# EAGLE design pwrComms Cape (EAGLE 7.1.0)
CNAME: Bristol Community College; CREVISION: v1r0; DESIGNER: J. Brian
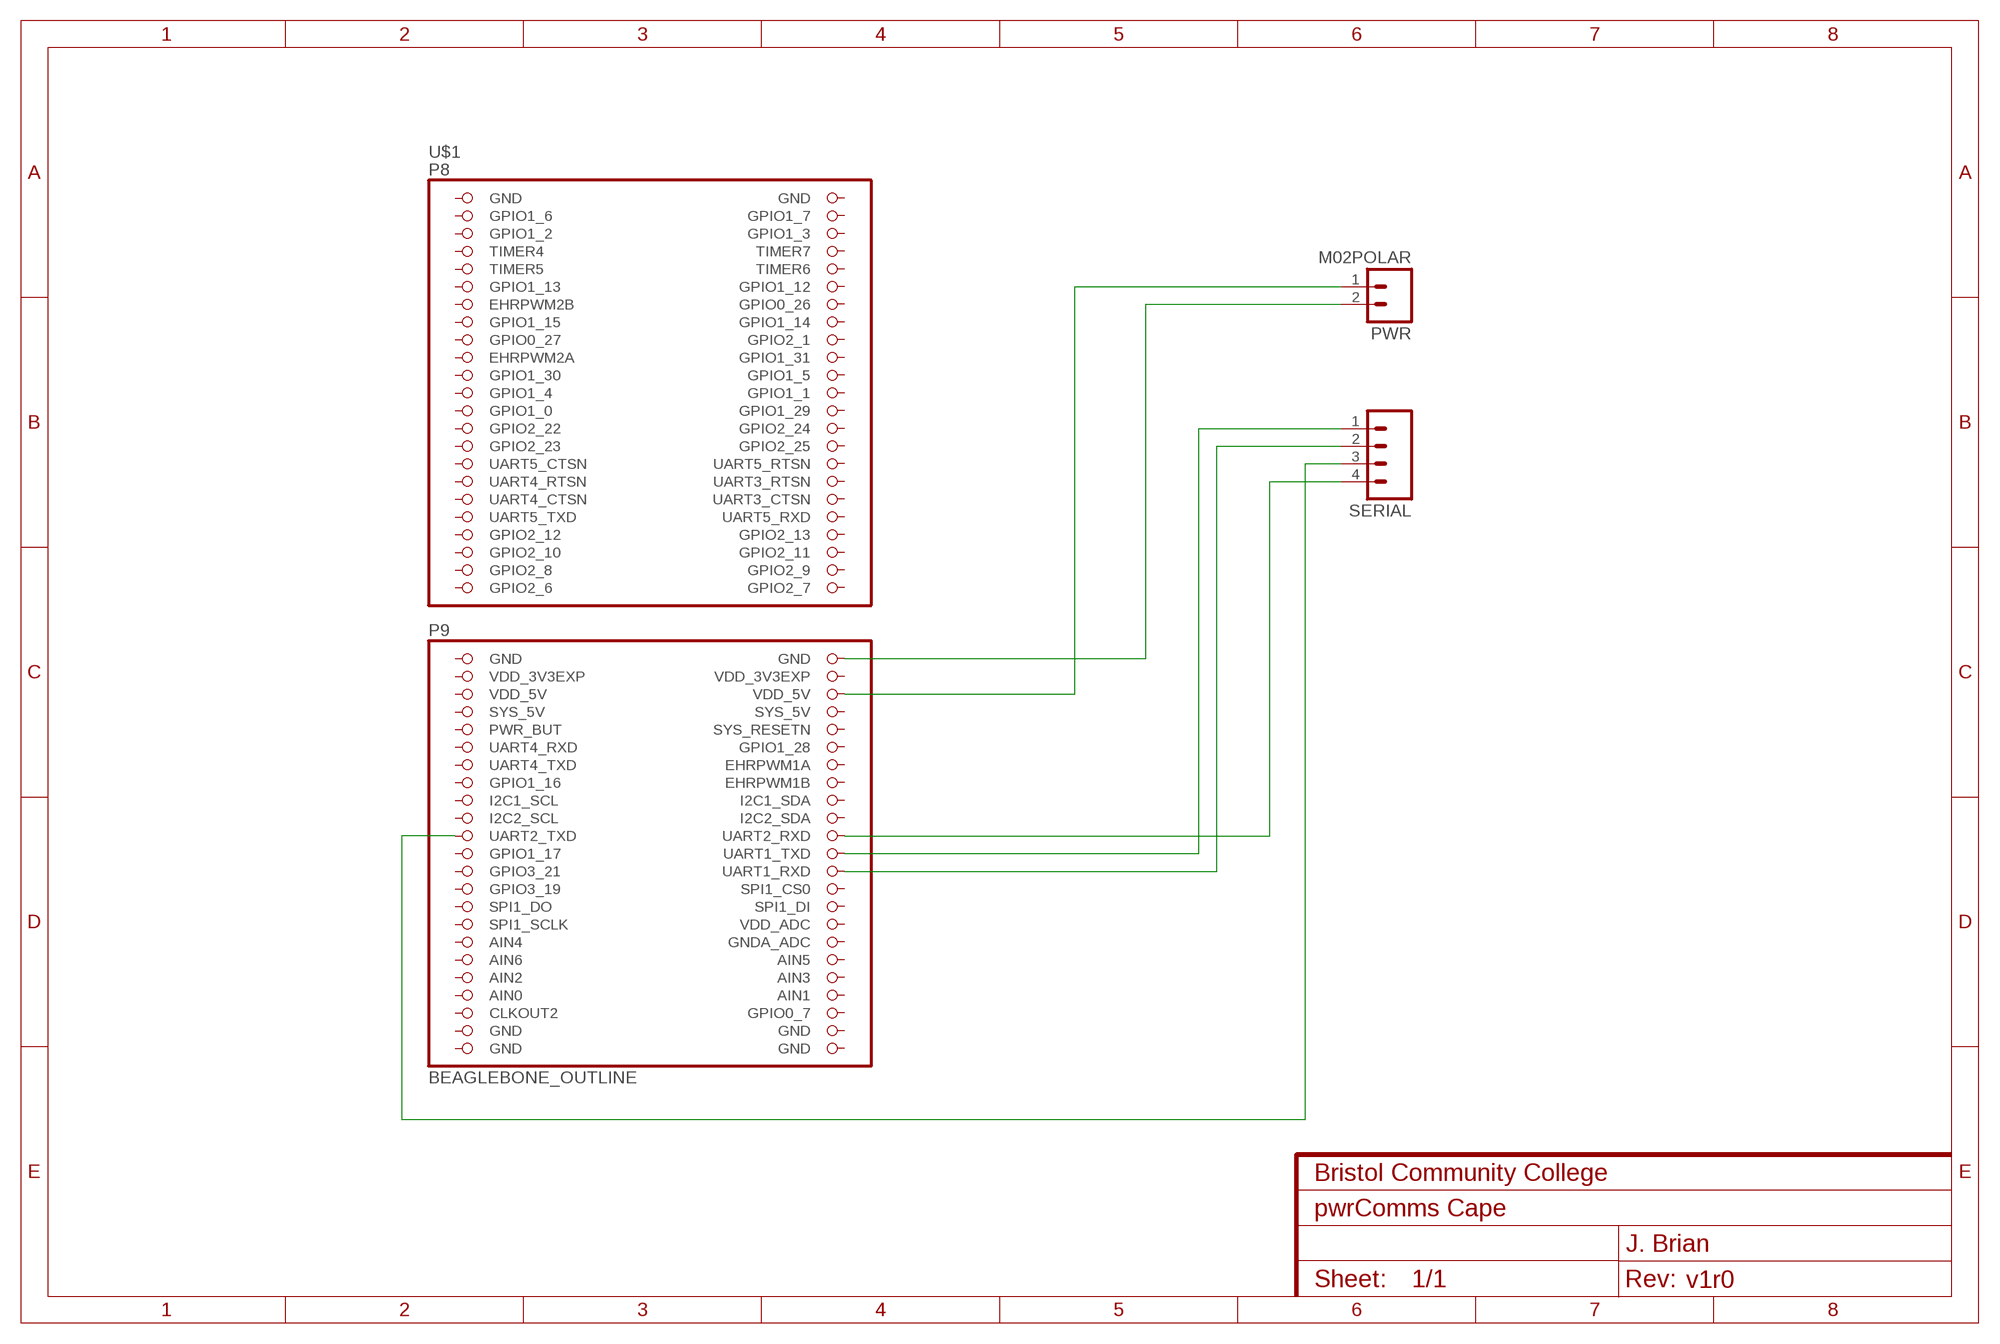
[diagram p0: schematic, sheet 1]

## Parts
PWR  M02POLAR  [MOLEX-1X2]
SERIAL  M04POLAR  [MOLEX-1X4]
U$1  BEAGLEBONE_OUTLINE  [BEAGLEBONE_SHIELD]

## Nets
GND: PWR.2 U$1.48(GND)
N$1: SERIAL.1 U$1.70(UART1_TXD)
N$3: SERIAL.4 U$1.68(UART2_RXD)
N$5: PWR.1 U$1.52(VDD_5V)
N$6: SERIAL.3 U$1.67(UART2_TXD)
N$7: SERIAL.2 U$1.72(UART1_RXD)
Unconnected: U$1.3(GPIO1_6) U$1.4(GPIO1_7) U$1.5(GPIO1_2) U$1.6(GPIO1_3) U$1.7(TIMER4) U$1.8(TIMER7) U$1.9(TIMER5) U$1.10(TIMER6) U$1.11(GPIO1_13) U$1.12(GPIO1_12) U$1.13(EHRPWM2B) U$1.14(GPIO0_26) U$1.15(GPIO1_15) U$1.16(GPIO1_14) U$1.17(GPIO0_27) U$1.18(GPIO2_1) U$1.19(EHRPWM2A) U$1.20(GPIO1_31) U$1.21(GPIO1_30) U$1.22(GPIO1_5) U$1.23(GPIO1_4) U$1.24(GPIO1_1) U$1.25(GPIO1_0) U$1.26(GPIO1_29) U$1.27(GPIO2_22) U$1.28(GPIO2_24) U$1.29(GPIO2_23) U$1.30(GPIO2_25) U$1.31(UART5_CTSN) U$1.32(UART5_RTSN) U$1.33(UART4_RTSN) U$1.34(UART3_RTSN) U$1.35(UART4_CTSN) U$1.36(UART3_CTSN) U$1.37(UART5_TXD) U$1.38(UART5_RXD) U$1.39(GPIO2_12) U$1.40(GPIO2_13) U$1.41(GPIO2_10) U$1.42(GPIO2_11) U$1.43(GPIO2_8) U$1.44(GPIO2_9) U$1.45(GPIO2_6) U$1.46(GPIO2_7) U$1.54(SYS_5V) U$1.55(PWR_BUT) U$1.56(SYS_RESETN) U$1.57(UART4_RXD) U$1.58(GPIO1_28) U$1.59(UART4_TXD) U$1.60(EHRPWM1A) U$1.61(GPIO1_16) U$1.62(EHRPWM1B) U$1.63(I2C1_SCL) U$1.64(I2C1_SDA) U$1.65(I2C2_SCL) U$1.66(I2C2_SDA) U$1.69(GPIO1_17) U$1.71(GPIO3_21) U$1.73(GPIO3_19) U$1.74(SPI1_CS0) U$1.75(SPI1_DO) U$1.76(SPI1_DI) U$1.77(SPI1_SCLK) U$1.78(VDD_ADC) U$1.79(AIN4) U$1.80(GNDA_ADC) U$1.81(AIN6) U$1.82(AIN5) U$1.83(AIN2) U$1.84(AIN3) U$1.86(AIN1) U$1.87(CLKOUT2) U$1.88(GPIO0_7)

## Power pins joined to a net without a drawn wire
AIN0: U$1.85(AIN0)
GND: U$1.1(GND) U$1.2(GND) U$1.47(GND) U$1.89(GND) U$1.90(GND) U$1.91(GND) U$1.92(GND)
SYS_5V: U$1.53(SYS_5V)
VDD_3V3EXP: U$1.49(VDD_3V3EXP) U$1.50(VDD_3V3EXP)
VDD_5V: U$1.51(VDD_5V)

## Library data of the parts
PWR = SparkFun-Connectors:M02: Standard 2-pin 0.1" header. Use with
SERIAL = SparkFun-Connectors:M04: Header 4 Standard 4-pin 0.1" header. Use with straight break away headers (SKU : PRT-00116), right angle break away headers (PRT-00553), swiss pins (PRT-00743), machine pins (PRT-00117), and female headers (PRT-00115). Molex polarized connector foot print use with SKU : PRT-08231 with associated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
U$1 = adafruit:BEAGLEBONE_OUTLINE: Should match A3 pinout - but not completely tested

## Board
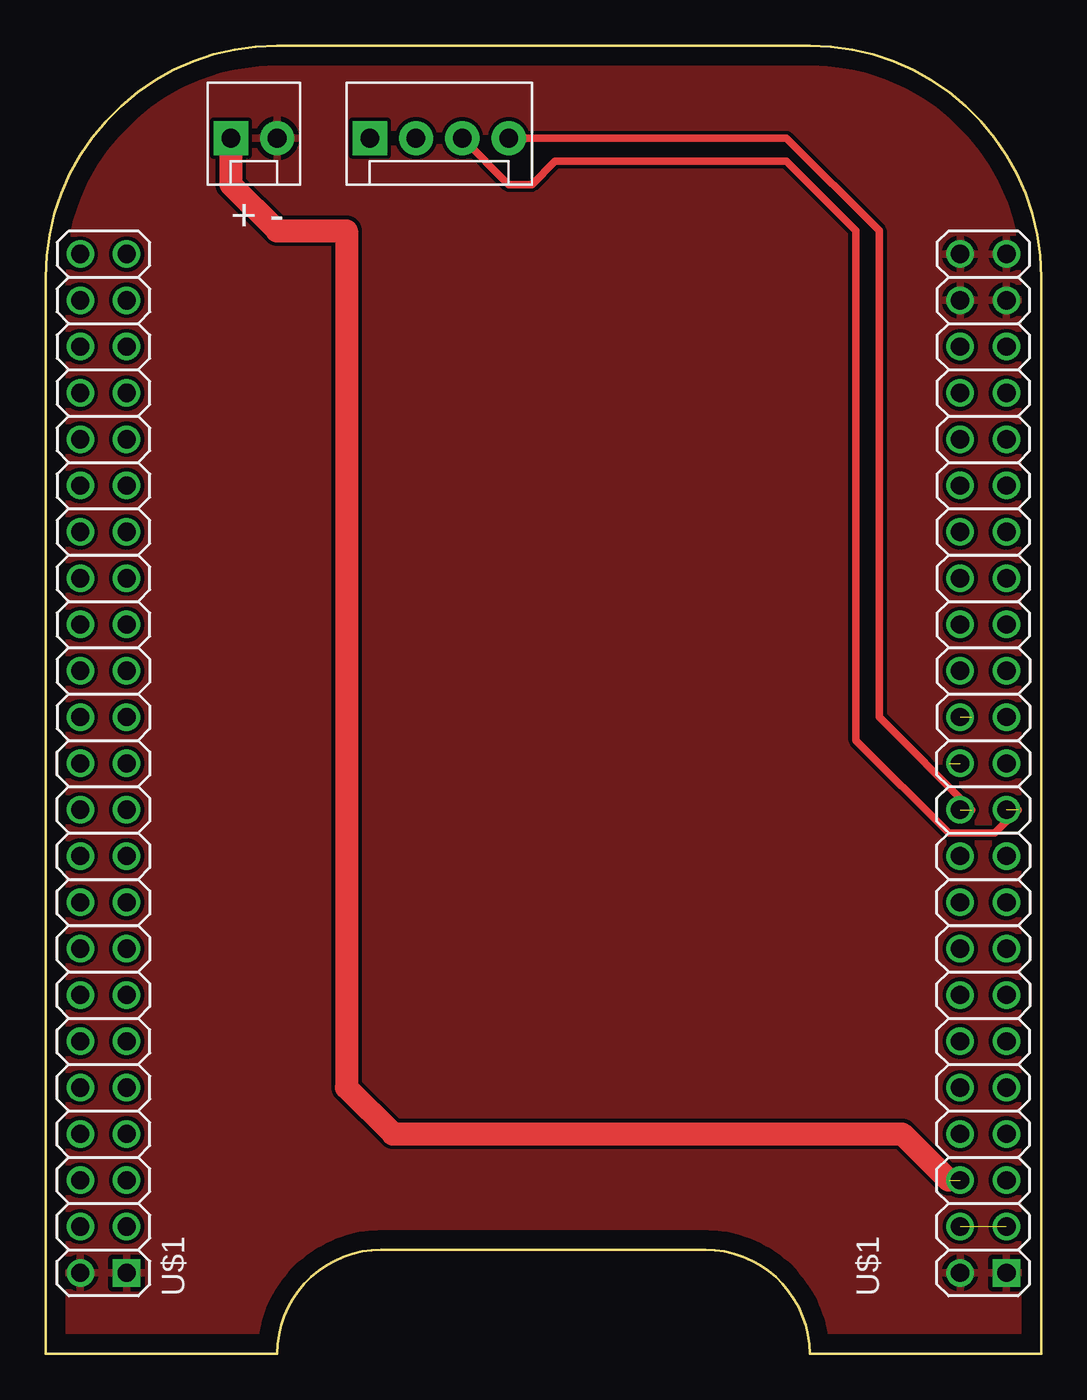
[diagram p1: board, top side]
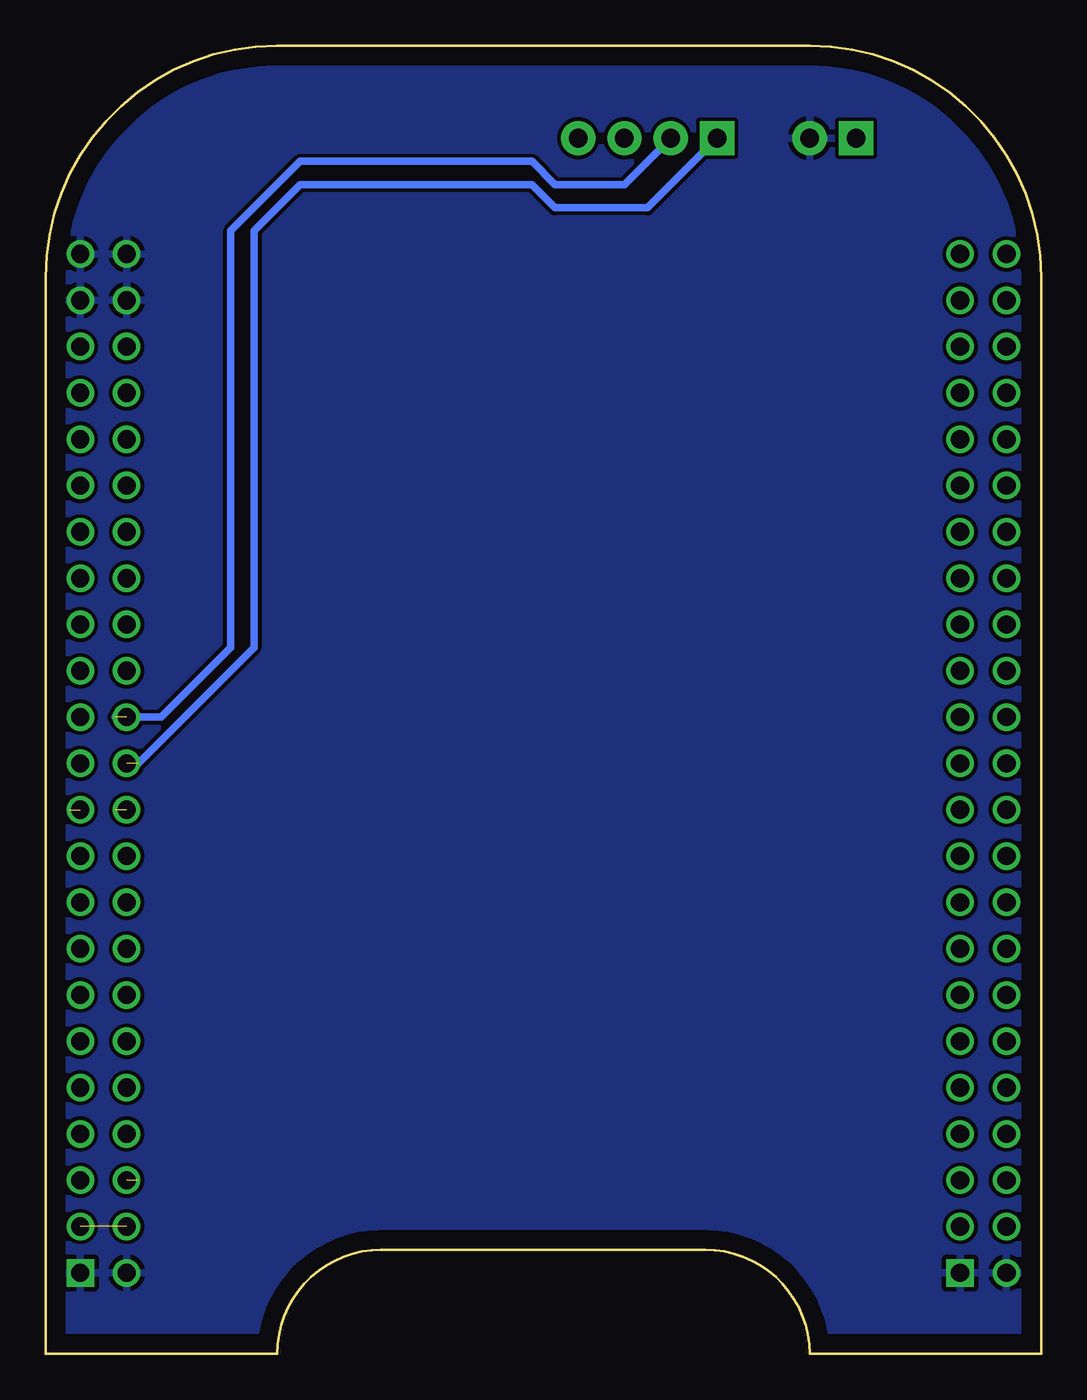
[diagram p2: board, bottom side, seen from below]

Size 54.61 x 71.75 mm. Coordinates in mm from the lower left corner, seen from the top.
Copper layers (1*16): Top 0.035mm / dielectric 1.5mm / Bottom 0.035mm
Design rules "default": minimum track width 10mil, minimum drill 24mil, track to track 8mil, track to pad 8mil, pad to pad 8mil, via to via 8mil, smd to smd 8mil, copper to edge 40mil, drill to drill 8mil, minimum pad ring 10mil, minimum via ring 8mil, stop-mask expansion 4mil, vias tented up to drill 0mil, thermal gap 10mil

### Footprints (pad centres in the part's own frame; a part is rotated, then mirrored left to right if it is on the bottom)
MOLEX-1X2 = drill 1.016 pad 1.88 square: 1 0,0 | drill 1.016 pad 1.88: 2 2.54,0
MOLEX-1X4 = drill 1.016 pad 1.88 square: 1 0,0 | drill 1.016 pad 1.88: 2 2.54,0; 3 5.08,0; 4 7.62,0
BEAGLEBONE_SHIELD = drill 1 square: 1 4.445,19.05; 47 52.705,19.05 | drill 1: 2 1.905,19.05; 3 4.445,21.59; 4 1.905,21.59; 5 4.445,24.13; 6 1.905,24.13; 7 4.445,26.67; 8 1.905,26.67; 9 4.445,29.21; 10 1.905,29.21; 11 4.445,31.75; 12 1.905,31.75; 13 4.445,34.29; 14 1.905,34.29; 15 4.445,36.83; 16 1.905,36.83; 17 4.445,39.37; 18 1.905,39.37; 19 4.445,41.91; 20 1.905,41.91; 21 4.445,44.45; 22 1.905,44.45; 23 4.445,46.99; 24 1.905,46.99; 25 4.445,49.53; 26 1.905,49.53; 27 4.445,52.07; 28 1.905,52.07; 29 4.445,54.61; 30 1.905,54.61; 31 4.445,57.15; 32 1.905,57.15; 33 4.445,59.69; 34 1.905,59.69; 35 4.445,62.23; 36 1.905,62.23; 37 4.445,64.77; 38 1.905,64.77; 39 4.445,67.31; 40 1.905,67.31; 41 4.445,69.85; 42 1.905,69.85; 43 4.445,72.39; 44 1.905,72.39; 45 4.445,74.93; 46 1.905,74.93; 48 50.165,19.05; 49 52.705,21.59; 50 50.165,21.59; 51 52.705,24.13; 52 50.165,24.13; 53 52.705,26.67; 54 50.165,26.67; 55 52.705,29.21; 56 50.165,29.21; 57 52.705,31.75; 58 50.165,31.75; 59 52.705,34.29; 60 50.165,34.29; 61 52.705,36.83; 62 50.165,36.83; 63 52.705,39.37; 64 50.165,39.37; 65 52.705,41.91; 66 50.165,41.91; 67 52.705,44.45; 68 50.165,44.45; 69 52.705,46.99; 70 50.165,46.99; 71 52.705,49.53; 72 50.165,49.53; 73 52.705,52.07; 74 50.165,52.07; 75 52.705,54.61; 76 50.165,54.61; 77 52.705,57.15; 78 50.165,57.15; 79 52.705,59.69; 80 50.165,59.69; 81 52.705,62.23; 82 50.165,62.23; 83 52.705,64.77; 84 50.165,64.77; 85 52.705,67.31; 86 50.165,67.31; 87 52.705,69.85; 88 50.165,69.85; 89 52.705,72.39; 90 50.165,72.39; 91 52.705,74.93; 92 50.165,74.93

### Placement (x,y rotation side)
PWR  10.16,66.67 0 top
SERIAL  17.78,66.67 0 top
U$1  0,-14.61 0 top

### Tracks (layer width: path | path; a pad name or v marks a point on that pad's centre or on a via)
GND
  pour Bottom: 41.91,71.75 11.43,71.75 arc90 0,60.33 0,0.63 12.7,0.63 arc-90 19.05,5.71 36.83,5.71 arc-90 41.91,0.63 54.61,0.63 54.61,59.05 arc90
  pour Top: 12.7,71.75 11.43,71.75 arc90 0,60.33 0,0.63 12.7,0.63 arc-90 17.78,5.71 36.83,5.71 arc-90 41.91,0.63 54.61,0.63 54.61,59.05 arc90 41.91,71.75
N$1  (1 unrouted)
  Bottom 0.406: SERIAL.1 21.59,62.86 26.67,62.86 27.94,64.13 40.64,64.13 43.18,61.59 43.18,38.73 49.53,32.39
N$3  (1 unrouted)
  Top 0.406: SERIAL.4 40.64,66.67 45.72,61.59 45.72,34.92 50.8,29.85
N$5  (1 unrouted)
  Top 1.27: PWR.1 10.16,64.13 12.7,61.59 16.51,61.59 16.51,14.61 19.05,12.07 46.99,12.07 49.53,9.52
N$6  (1 unrouted)
  Top 0.406: 53.34,29.85 52.07,28.57 49.53,28.57 44.45,33.66 44.45,61.59 40.64,65.41 27.94,65.41 26.67,64.13 25.4,64.13 SERIAL.3
N$7  (1 unrouted)
  Bottom 0.406: 50.8,34.92 48.26,34.92 44.45,38.73 44.45,61.59 40.64,65.41 27.94,65.41 26.67,64.13 22.86,64.13 SERIAL.2
VDD_3V3EXP  (1 unrouted)

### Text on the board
tNames: + -

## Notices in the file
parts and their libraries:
SparkFun-Aesthetics: Licensing: Creative Commons ShareAlike 4.0 International - https://creativecommons.org/licenses/by-sa/4.0
